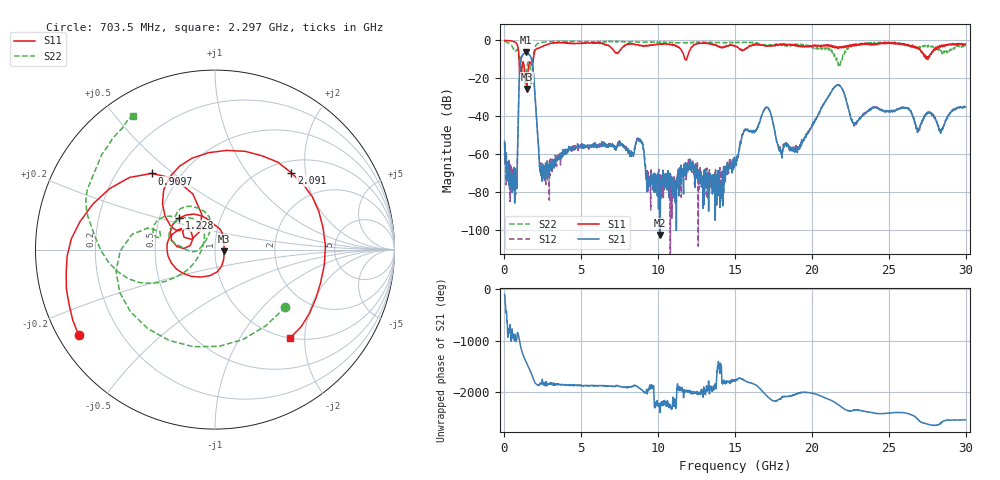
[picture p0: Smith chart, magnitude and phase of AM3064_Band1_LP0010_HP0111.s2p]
# Hz S DB R 50.0
!freq dBS11 angS11 dBS21 angS21 dBS12 angS12 dBS22 angS22
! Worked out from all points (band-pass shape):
!   1600 points, 10 MHz to 29.98 GHz, reference 50 ohm
!   highest |S21| = -6.24 dB at 1.378 GHz (marker M1); lowest = -102.6 dB at 10.13 GHz (marker M2)
!   |S21| within 3 dB of the highest: 1.101 GHz to 1.733 GHz (632.1 MHz wide, 44.6 % of centre)
!   lowest |S11| = -25.5 dB at 1.453 GHz (marker M3), VSWR 1.11, Z = 55.5 - j1.09 ohm
!   |S11| at or under -10 dB: 949.4 MHz to 1.878 GHz (928.7 MHz wide, 65.7 % of centre); 11.76 GHz to 11.84 GHz (87.48 MHz wide, 0.741 % of centre); 27.5278 GHz to 27.54639 GHz (18.59 MHz wide, 0.0675 % of centre)
!   |S22| runs from -23.1 to -0.2 dB; largest |S21 - S12| = 0.0061
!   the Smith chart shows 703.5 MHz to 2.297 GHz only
!   S11 on the Smith chart (normalised r, x): 703.5 MHz: 0.06, -0.29; 909.7 MHz: 0.35, +0.42; 1.228 GHz: 0.63, +0.24; 2.091 GHz: 1.24, +1.67; 2.297 GHz: 1.01, -1.70
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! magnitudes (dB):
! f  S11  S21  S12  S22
! 10 MHz  0.0  -53.3  -53.6  -0.2
! 703.5 MHz  -0.9  -69.2  -68.3  -5.9
! 909.7 MHz  -5.2  -36.3  -36.1  -6.6
! 1.228 GHz  -11.5  -7.2  -7.2  -12.1
! 1.378 GHz  -18.7  -6.2  -6.2  -19.9
! 1.453 GHz  -25.5  -6.4  -6.3  -14.7
! 1.791 GHz  -13.1  -11.0  -10.9  -17.6
! 2.091 GHz  -4.4  -41.7  -41.2  -2.1
! 2.297 GHz  -3.8  -65.6  -64.3  -1.2
! 5.015 GHz  -1.3  -55.3  -56.5  -0.7
! 8.763 GHz  -2.8  -53.1  -52.5  -1.0
! 9.363 GHz  -2.8  -73.1  -71.4  -0.9
! 10 GHz  -2.0  -69.7  -72.3  -0.9
! 10.13 GHz  -1.8  -102.6  -70.9  -1.0
! 15 GHz  -3.0  -64.4  -63.7  -1.3
! 17.01 GHz  -3.1  -35.2  -35.3  -2.5
! 17.97 GHz  -2.4  -58.6  -58.6  -2.2
! 19.99 GHz  -3.2  -45.3  -45.5  -3.4
! 21.68 GHz  -4.3  -23.4  -23.5  -11.3
! 22.75 GHz  -3.0  -43.6  -44.5  -1.9
! 25 GHz  -1.1  -37.2  -37.4  -1.2
! 29.98 GHz  -1.9  -35.1  -35.1  -3.2
